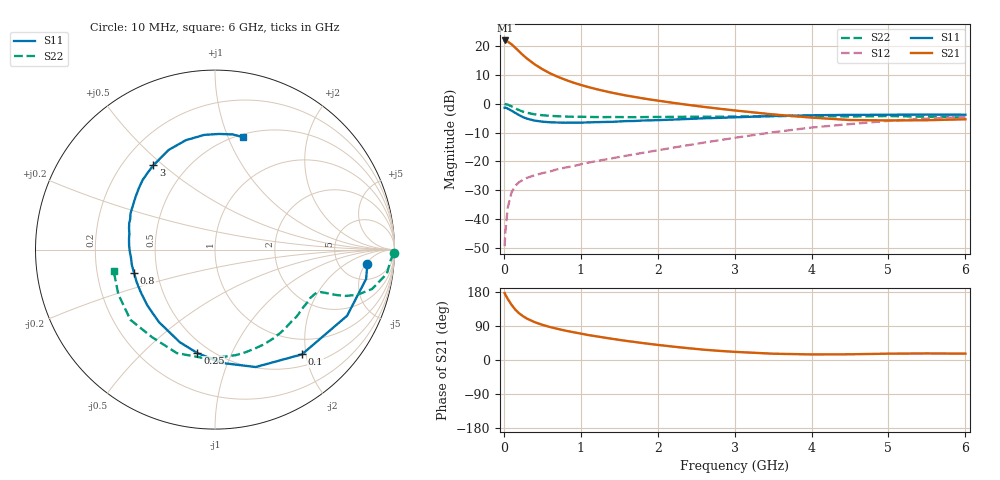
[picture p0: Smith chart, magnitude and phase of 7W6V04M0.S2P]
! Infineon Technologies  Discrete & RF Semiconductors
! BFS17W
! Si NPN RF Bipolar Junction Transistor in SOT323
! VCE = 6 V  IC = 4 mA
! Common Emitter S-Parameters:  August  1999
# GHz  S  MA  R  50
!  f  S11  S21  S12  S22
! GHz  MAG  ANG  MAG  ANG  MAG  ANG  MAG  ANG
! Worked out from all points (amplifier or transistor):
!   36 points, 10 MHz to 6 GHz, reference 50 ohm
!   highest |S21| = 21.9 dB at 20 MHz (marker M1)
!   |S21| within 3 dB of that: start of sweep to 167.4 MHz
!   unconditionally stable (mu >= 1): 631 MHz to 2.545 GHz; 4.8 GHz to end of sweep
!   at 250 MHz: K = 0.52, MSG = 21.6 dB, |S12| = -26.4 dB
!   at 1.4 GHz: K = 1.24, MAG = 8.5 dB, |S12| = -19.0 dB
!   at 6 GHz: K = 1.07, MAG = -2.0 dB, |S12| = -4.5 dB
!   S11 on the Smith chart (normalised r, x): 10 MHz: 9, -5; 100 MHz: 0.70, -1.93; 250 MHz: 0.43, -0.75; 800 MHz: 0.37, -0.12; 3 GHz: 0.33, +0.46; 6 GHz: 0.53, +1.14
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0.01  0.8527 -5.3  12.48 176.7  0.0034 82.4  0.997 -1.2
0.02  0.8576 -11.0  12.49 172.4  0.0061 84.5  0.9813 -3.3
0.05  0.8231 -26.6  11.96 161.4  0.0156 77.3  0.9668 -8.0
0.1  0.7586 -50.3  10.73 145.7  0.029 66.0  0.902 -14.1
0.15  0.6924 -70.9  9.31 132.7  0.038 57.7  0.8302 -17.7
0.2  0.6322 -86.7  8.036 123.0  0.0438 54.2  0.7726 -19.5
0.25  0.5846 -99.7  6.938 115.5  0.0481 50.0  0.728 -20.4
0.3  0.5521 -110.8  6.083 109.3  0.0519 48.8  0.6975 -20.9
0.4  0.5104 -127.8  4.824 99.9  0.0577 47.8  0.6545 -21.5
0.5  0.489 -140.2  3.978 92.9  0.0626 48.7  0.6323 -22.0
0.6  0.4772 -149.8  3.369 87.0  0.067 50.3  0.6167 -22.9
0.8  0.4692 -164.1  2.601 77.5  0.0783 53.8  0.6007 -25.7
0.9  0.4713 -169.6  2.33 73.5  0.0829 55.5  0.5948 -27.2
1.1  0.4754 -179.2  1.943 65.8  0.0954 58.1  0.5905 -30.9
1.3  0.4832 172.6  1.67 59.3  0.1069 60.9  0.5862 -35.2
1.6  0.5006 162.7  1.381 50.2  0.126 63.9  0.5849 -41.8
2.2  0.5315 146.3  1.037 35.3  0.1732 68.1  0.5921 -57.0
3  0.5818 126.2  0.765 21.5  0.2566 68.2  0.5994 -78.8
3.5  0.6124 114.9  0.653 16.6  0.3207 65.2  0.6101 -93.7
4.5  0.642 95.3  0.522 15.1  0.4437 53.5  0.6009 -125.7
5.5  0.6493 81.2  0.518 17.3  0.5516 40.3  0.5934 -155.2
6  0.6453 75.8  0.538 16.8  0.5944 33.9  0.5771 -168.3
